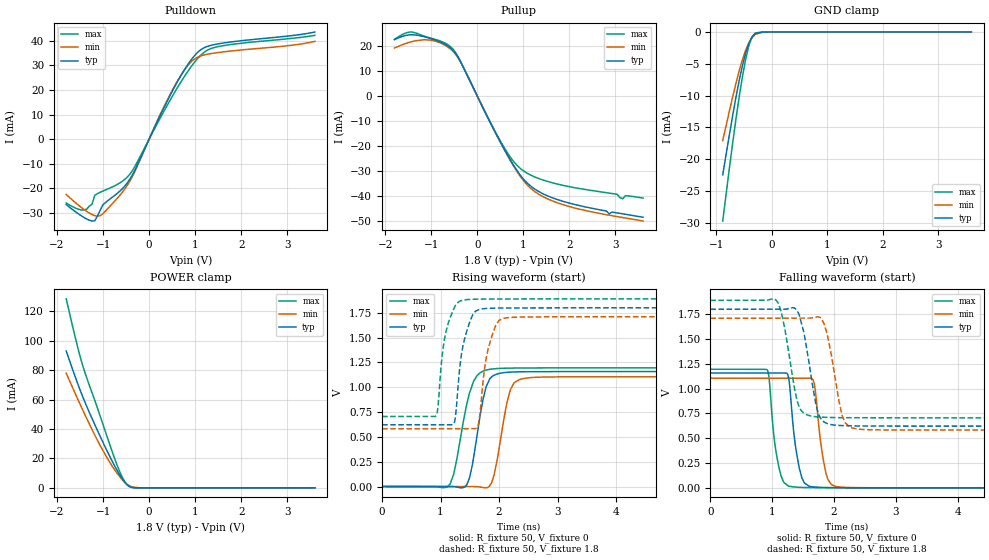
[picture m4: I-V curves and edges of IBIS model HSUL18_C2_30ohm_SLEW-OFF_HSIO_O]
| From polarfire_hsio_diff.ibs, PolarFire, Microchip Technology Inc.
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|   Model HSUL18_C2_30ohm_SLEW-OFF_HSIO_O
[Model]   HSUL18_C2_30ohm_SLEW-OFF_HSIO_O
Model_type   Output
Polarity   Non-Inverting
Enable   Active-High
Vmeas =   0.9
Cref =   5p
Rref =   50
Vref =   0.9
|   typ   min   max
C_comp_pullup   1.335e-12   1.335e-12   1.380e-12
C_comp_pulldown  1.335e-12   1.335e-12   1.380e-12
[Temperature Range]  25C   100C   -40C
[Voltage Range]  1.8   1.71   1.89
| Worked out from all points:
|   slope of the pulldown table from 0 to 0.27 V, typ, clamps not added: 25 ohm
|   slope of the pullup table from 0 to 0.27 V, typ, clamps not added: 26.6 ohm
|   GND clamp passes 1 mA (typ) near -0.37 V on its own axis
|   POWER clamp passes 1 mA (typ) near -0.43 V on its own axis
|   rising waveform, R_fixture 50, V_fixture 0: 20-80 % time 199ps typ, 203ps min, 238ps max; typ from 0 V to 1.16 V
|   rising waveform, R_fixture 50, V_fixture 1.8: 20-80 % time 168ps typ, 176ps min, 161ps max; typ from 0.622 V to 1.8 V
|   falling waveform, R_fixture 50, V_fixture 0: 20-80 % time 131ps typ, 131ps min, 129ps max; typ from 1.16 V to 0 V
|   falling waveform, R_fixture 50, V_fixture 1.8: 20-80 % time 188ps typ, 193ps min, 193ps max; typ from 1.8 V to 0.622 V
[GND Clamp]
| Voltage   I(typ)   I(min)   I(max)
-885.9mV  -22.44mA   -17.06mA   -29.71mA
-708.7mV  -13.24mA   -10.28mA   -17.6mA
-649.7mV  -10.37mA   -8.138mA   -13.83mA
-590.6mV  -7.705mA   -6.148mA   -10.3mA
-531.6mV  -5.322mA   -4.371mA   -7.074mA
-472.5mV  -3.308mA   -2.865mA   -4.286mA
-413.4mV  -1.757mA   -1.684mA   -2.101mA
-354.4mV  -739.5uA   -855.1uA   -713.7uA
-295.3mV  -232.3uA   -363.2uA   -148.3uA
-177.2mV  -12.01uA   -39.02uA   -3.177uA
-59.06mV  -489.8nA   -2.616uA   -234.3nA
3.6V      0A         0A         0A
[POWER Clamp]
| Voltage   I(typ)   I(min)   I(max)
-1.8V     93.11mA    78.02mA    128.6mA
-1.595V   74.64mA    63.48mA    101.1mA
-1.477V   64.73mA    55.33mA    86.9mA
-1.417V   60.07mA    51.32mA    80.62mA
-1.063V   35.01mA    28.82mA    48.84mA
-885.9mV  23.32mA    19.01mA    32.31mA
-708.7mV  12.62mA    10.48mA    16.53mA
-590.6mV  6.476mA    5.751mA    7.626mA
-472.5mV  1.932mA    2.149mA    1.873mA
-354.4mV  154uA      469.9uA    209.6uA
-236.2mV  4.969uA    79.11uA    56.46uA
3.6V      0A         0A         0A
[Pullup]
| Voltage   I(typ)   I(min)   I(max)
-1.8V     22.73mA    19.34mA    22.85mA
-1.417V   24.7mA     21.94mA    25.78mA
-945mV    22.75mA    22.24mA    22.99mA
-531.6mV  18.47mA    18.08mA    18.92mA
-354.4mV  13.52mA    13.37mA    13.55mA
618.8mV   -22.42mA   -22.61mA   -21.73mA
900mV     -30.89mA   -31.35mA   -28.46mA
1.238V    -37.19mA   -38.16mA   -32.37mA
1.977V    -42.84mA   -44.21mA   -36.26mA
3.04V     -46.88mA   -48.37mA   -39.41mA
3.158V    -47.25mA   -48.74mA   -41.17mA
3.6V      -48.65mA   -50.14mA   -40.92mA
[Pulldown]
| Voltage   I(typ)   I(min)   I(max)
-1.8V     -26.65mA   -22.54mA   -26mA
-1.477V   -31.16mA   -27.74mA   -28.82mA
-1.24V    -33.33mA   -30.69mA   -26.51mA
-1.181V   -33.27mA   -31.14mA   -22.88mA
-1.004V   -26.72mA   -30.4mA    -21.14mA
-649.7mV  -21.41mA   -23.19mA   -17.99mA
-413.4mV  -16.19mA   -16.93mA   -14.15mA
562.5mV   21.56mA    21.92mA    19.3mA
843.8mV   30.43mA    30.03mA    27.65mA
1.125V    36.41mA    33.87mA    34.2mA
1.575V    39mA       35.41mA    37.92mA
3.6V      43.57mA    39.78mA    42.22mA
[Ramp]
dV/dt_r   0.694964/0.198754n  0.663492/0.202789n  0.717208/0.238114n
dV/dt_f   0.707015/0.188312n  0.676821/0.193484n  0.710764/0.192575n
R_load = 50
[Rising Waveform]
R_fixture = 50
V_fixture = 0
V_fixture_min = 0
V_fixture_max = 0
| Time   V(typ)   V(min)   V(max)
0s        2.204uV    2.277uV    4.182uV
1.113ns   -358.9uV   -426.8uV   -4.605mV
1.224ns   -1.387mV   -469.6uV   121.9mV
1.41ns    -6.599mV   -541.3uV   715.9mV
1.565ns   291.7mV    -601.1uV   1.06V
1.787ns   1.014V     -12.16mV   1.174V
1.915ns   1.12V      116.1mV    1.185V
2.194ns   1.152V     975.1mV    1.193V
2.407ns   1.156V     1.086V     1.194V
10ns      1.158V     1.106V     1.195V
[Rising Waveform]
R_fixture = 50
V_fixture = 1.8
V_fixture_min = 1.71
V_fixture_max = 1.89
| Time   V(typ)   V(min)   V(max)
0s        621.6mV    581.9mV    705.4mV
925ps     622mV      582.3mV    714.4mV
959ps     622mV      582.3mV    819.8mV
1.068ns   622.1mV    582.3mV    1.487V
1.233ns   641.6mV    582.4mV    1.797V
1.392ns   1.44V      582.4mV    1.878V
1.64ns    1.777V     613.1mV    1.887V
1.818ns   1.794V     1.395V     1.888V
2.066ns   1.798V     1.692V     1.889V
10ns      1.8V       1.71V      1.89V
[Falling Waveform]
R_fixture = 50
V_fixture = 0
V_fixture_min = 0
V_fixture_max = 0
| Time   V(typ)   V(min)   V(max)
0s        1.158V     1.106V     1.195V
921ps     1.158V     1.105V     1.188V
1.07ns    1.157V     1.105V     336.8mV
1.263ns   1.116V     1.105V     17.95mV
1.439ns   199.9mV    1.105V     5.075mV
1.605ns   14.2mV     1.105V     2.464mV
1.681ns   8.753mV    1.052V     2.085mV
1.872ns   3.115mV    143.1mV    1.431mV
2.038ns   1.834mV    12.45mV    1.176mV
10ns      3.134uV    3.559uV    4.559uV
[Falling Waveform]
R_fixture = 50
V_fixture = 1.8
V_fixture_min = 1.71
V_fixture_max = 1.89
| Time   V(typ)   V(min)   V(max)
0s        1.8V       1.71V      1.89V
1.068ns   1.801V     1.711V     1.889V
1.147ns   1.801V     1.711V     1.775V
1.435ns   1.749V     1.711V     822.3mV
1.634ns   1.109V     1.712V     723.4mV
1.794ns   689.2mV    1.705V     712.8mV
1.89ns    648.5mV    1.551V     710.1mV
2.134ns   627.4mV    726.3mV    707.4mV
2.302ns   624.6mV    602.5mV    706.8mV
10ns      621.6mV    581.9mV    705.4mV
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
